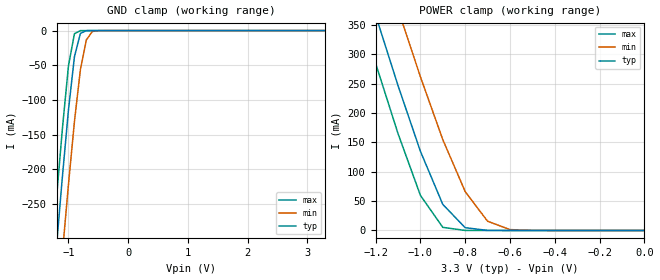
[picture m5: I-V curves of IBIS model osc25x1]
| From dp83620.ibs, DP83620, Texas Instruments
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|   Model osc25x1
[Model]   osc25x1
Model_type   Input
Polarity   Inverting
Enable   Active-High
Vinl = 0.8000V
Vinh = 2.0000V
C_comp   1.0000pF   1.0000pF   1.0000pF
[Temperature Range]   25.0000   0.1250k   -40.0000
[Voltage Range]   3.3000V   3.0000V   3.6000V
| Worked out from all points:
|   GND clamp passes 1 mA (typ) near -0.72 V on its own axis
|   POWER clamp passes 1 mA (typ) near -0.72 V on its own axis
[GND_clamp]
| voltage   I(typ)   I(min)   I(max)
-3.3V     -2.622A    -2.694A    -2.579A
-1.3V     -414.8mA   -523mA     -346.4mA
-1.2V     -310.3mA   -419.8mA   -240.9mA
-1.1V     -208.9mA   -318.8mA   -139.7mA
-1V       -114.1mA   -221.5mA   -50.66mA
-900mV    -37.58mA   -131mA     -4.515mA
-800mV    -4.019mA   -56.03mA   -47.48uA
-700mV    -108.1uA   -13.33mA   -2.355uA
-600mV    -3.685uA   -1.282mA   -1.753uA
-400mV    -1.001uA   -4.899uA   -1.167uA
3.3V      8.25uA     7.477uA    9.629uA
[POWER_clamp]
| voltage   I(typ)   I(min)   I(max)
-3.3V     3.1A       3.186A     3.05A
-1.3V     490.5mA    618.5mA    409.7mA
-1.2V     366.9mA    496.4mA    284.9mA
-1.1V     247mA      377mA      165.2mA
-1V       135mA      261.9mA    59.9mA
-900mV    44.44mA    154.8mA    5.346mA
-800mV    4.759mA    66.25mA    66.21uA
-700mV    135.7uA    15.76mA    12.92uA
-600mV    12.33uA    1.522mA    12.26uA
-500mV    9.553uA    95.08uA    11.96uA
0V        8.25uA     6.563uA    10.5uA
